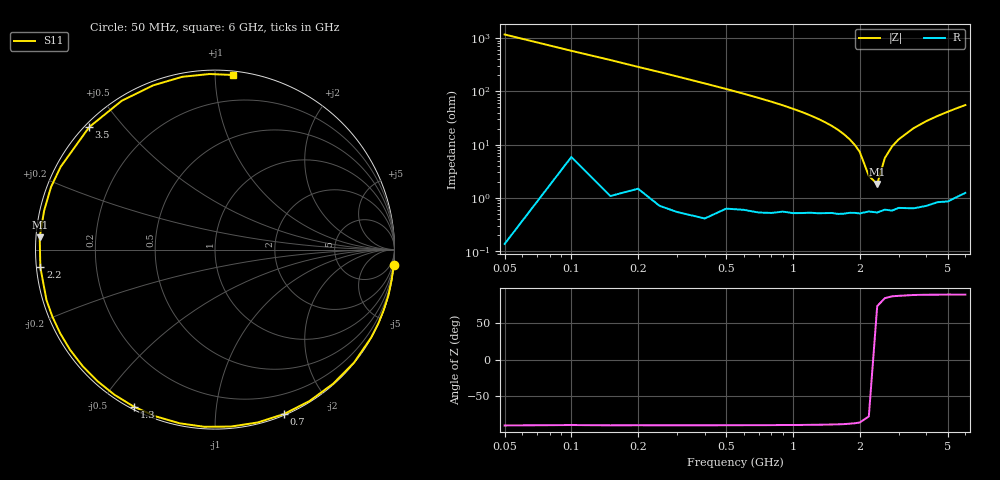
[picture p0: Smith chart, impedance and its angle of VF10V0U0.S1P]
! Infineon Technologies  Discrete & RF Semiconductors
! BBY 58-03
! Si Tuning Diode in SOD323
! VR = 10 V
! S-Parameters:  June  1999
# GHz  S  MA  R  50
!  f  S11
! GHz  MAG  ANG
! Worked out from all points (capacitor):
!   34 points, 50 MHz to 6 GHz, reference 50 ohm
!   read as one part to ground: C = 2.73 pF near 50 MHz
!   lowest |Z| = 1.83 ohm at 2.4 GHz (marker M1)
!   series resonance near 2.318 GHz, so ESL is about 1.7 nH
!   S11 on the Smith chart (normalised r, x): 50 MHz: 0, -23; 700 MHz: 0.01, -1.51; 1.3 GHz: 0.01, -0.61; 2.2 GHz: 0.01, -0.05; 3.5 GHz: 0.01, +0.41; 6 GHz: 0.02, +1.11
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0.05  1 -4.9
0.15  0.9993 -14.7
0.3  0.9986 -29.4
0.4  0.9982 -39.1
0.5  0.9958 -48.6
0.6  0.9944 -58.0
0.7  0.9935 -67.2
0.8  0.9921 -76.1
0.9  0.99 -84.8
1  0.9891 -93.4
1.1  0.9876 -101.6
1.3  0.9851 -117.3
1.4  0.9839 -124.7
1.6  0.9826 -138.6
1.7  0.9817 -145.3
1.9  0.98 -157.6
2  0.9802 -163.3
2.2  0.978 -174.2
2.4  0.979 176.0
2.6  0.9765 167.2
2.8  0.9779 159.1
3  0.9758 151.8
3.5  0.9784 135.8
4  0.9785 122.1
4.5  0.9777 110.6
5  0.9798 100.7
5.5  0.9787 91.8
6  0.9779 84.2
